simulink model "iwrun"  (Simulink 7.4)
settings: Solver=ode45  StartTime=0  StopTime=5  MaxStep=5e-4  RelTol=1e-3
libraries: mrlib x1

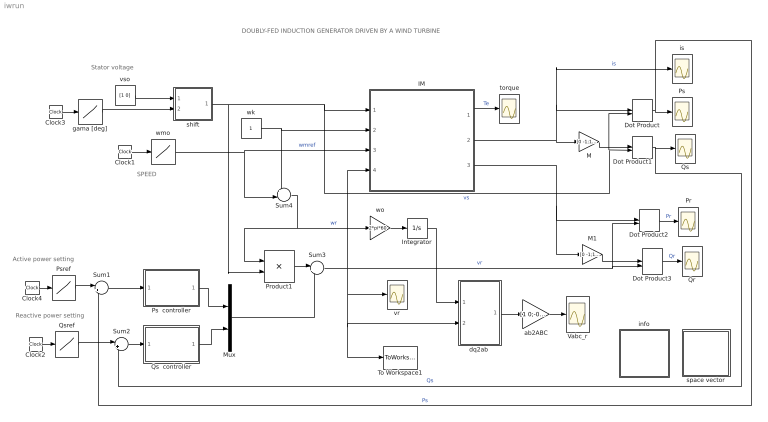
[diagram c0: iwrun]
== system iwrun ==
  note: DOUBLY-FED INDUCTION GENERATOR DRIVEN BY A WIND TURBINE
  note: SPEED
  note: Reactive power setting
  note: Active power setting
  note: Stator voltage
  Clock{1..4} (4 alike) : Clock
  Dot Product{,1..3} (4 alike) : DotProduct  OutDataType=fixdt(1, 16)  OutScaling=2^-10
  IM : Subsystem  mask{Rs=0.01, Lsl=0.1, Rr=0.02, Lm=5, Lrl=0.1, wo=2*pi*60}
      mask prompts: Rs "Stator resistance [pu]"; Lsl "Stator leakage inductance [pu]"; Rr "Rotor resistance [pu]"; Lm "Magnetizing inductance [pu]"; Lrl "Rotor leakage inductance [pu]"; wo "base frequency [rad/s]"
  Integrator : Integrator
  M : Gain  Gain=[0 -1;1 0]  Multiplication=Matrix(K*u)  ParameterDataType=sfix(16)  ParameterScaling=2^0  OutDataType=sfix(16)  OutScaling=2^0
  M1 : Gain  Gain=[0 -1;1 0]  Multiplication=Matrix(K*u)  ParameterDataType=sfix(16)  ParameterScaling=2^0  OutDataType=sfix(16)  OutScaling=2^0
  Mux : Mux  Inputs=2
  Pr : Scope
  Product1 : Product  OutDataType=sfix(16)  OutScaling=2^0
  Ps : Scope
  Ps  controller : Subsystem  mask{Kp=.1, Ki=10, sat=3}
      mask prompts: Kp "Proportional gain (Kp)"; Ki "Integral gain (Ki)"; sat "Saturation limit [pu]"
      mask help: Proportional-Integral Speed Controller
  Psref : Lookup  InputValues=[0 2 2.01 10 ]  Table=[0 0 -1 -1]  OutDataType=sfix(16)  OutScaling=2^0
  Qr : Scope
  Qs : Scope
  Qs  controller : Subsystem  mask{Kp=.1, Ki=10, sat=1000}
      mask prompts: Kp "Proportional gain (Kp)"; Ki "Integral gain (Ki)"; sat "Saturation limit [pu]"
      mask help: Proportional-Integral Speed Controller
  Qsref : Lookup  InputValues=[0 3 3.01 30 ]  Table=[0 0 .5 .5]  OutDataType=sfix(16)  OutScaling=2^0
  Sum1 : Sum  Inputs=|+-  OutDataType=sfix(16)  OutScaling=2^0
  Sum2 : Sum  Inputs=|++  OutDataType=sfix(16)  OutScaling=2^0
  Sum3 : Sum  Inputs=|+-  OutDataType=sfix(16)  OutScaling=2^0
  Sum4 : Sum  Inputs=+-|  OutDataType=sfix(16)  OutScaling=2^0
  To Workspace1 : ToWorkspace  VariableName=vro  SampleTime=-1  SaveFormat=Array
  Vabc_r : Scope
  ab2ABC : Gain  Gain=[1 0;-0.5 sqrt(3)/2;-0.5 -sqrt(3)/2]  Multiplication=Matrix(K*u)  ParameterDataType=sfix(16)  ParameterScaling=2^0  OutDataType=sfix(16)  OutScaling=2^0
  "dq2ab " : Subsystem
  gama [deg] : Lookup  InputValues="[0  1 1.01 5]"  Table=[0 0 10 10]  OutDataType=sfix(16)  OutScaling=2^0
  info : Subsystem
  is : Scope
  shift : Subsystem
  space vector : Subsystem
  torque : Scope
  vr : Scope
  vso : Constant  Value=[1 0]  OutDataType=sfix(16)  OutScaling=2^0
  wk : Constant  OutDataType=sfix(16)  OutScaling=2^0
  wmo : Lookup  InputValues=[0 4 4.01 20 ]  Table=[.7 .7 1.3 1.3]  OutDataType=sfix(16)  OutScaling=2^0
  wo : Gain  Gain=2*pi*60  ParameterDataType=sfix(16)  ParameterScaling=2^0  OutDataType=sfix(16)  OutScaling=2^0
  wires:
  shift/1(vs) -> IM/1(vs), Dot Product/2, Dot Product1/2, Product1/2  "vs"
  wk/1 -> IM/2(wk), Sum4/1
  Dot Product/1 -> Ps/1, Sum1/2  "Ps"
  M/1 -> Dot Product1/1
  Dot Product1/1 -> Qs/1, Sum2/2  "Qs"
  IM/2(is) -> M/1, Dot Product/1, is/1  "is"
  Dot Product2/1 -> Pr/1  "Pr"
  M1/1 -> Dot Product3/1
  Dot Product3/1 -> Qr/1  "Qr"
  IM/3(ir) -> M1/1, Dot Product2/1
  Clock1/1 -> wmo/1
  wmo/1 -> IM/3(wm), Sum4/2  "wmref"
  IM/1(Te) -> torque/1  "Te"
  Qs  controller/1(Vsqer) -> Mux/2
  Sum2/1 -> Qs  controller/1(Qser)
  Sum1/1 -> Ps  controller/1(Pser)
  Ps  controller/1(Vsder) -> Mux/1
  Sum4/1 -> Product1/1, wo/1  "wr"
  Product1/1 -> Sum3/1
  Sum3/1 -> IM/4(vr), Dot Product3/2, Dot Product2/2, vr/1, "dq2ab "/2(dq), To Workspace1/1  "vr"
  Clock4/1 -> Psref/1
  Psref/1 -> Sum1/1
  Clock2/1 -> Qsref/1
  Qsref/1 -> Sum2/1
  Clock3/1 -> gama [deg]/1
  vso/1 -> shift/1(vso)
  gama [deg]/1 -> shift/2(gama)
  "dq2ab "/1(ab) -> ab2ABC/1
  ab2ABC/1 -> Vabc_r/1
  wo/1 -> Integrator/1
  Integrator/1 -> "dq2ab "/1(thetar)
  Mux/1 -> Sum3/2

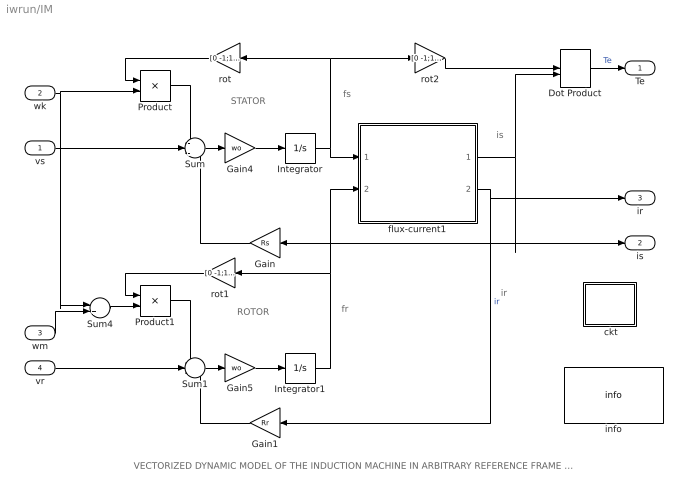
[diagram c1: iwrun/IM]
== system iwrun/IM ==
  note: ROTOR
  note: STATOR
  note: fs
  note: fr
  note: is
  note: VECTORIZED DYNAMIC MODEL OF THE INDUCTION MACHINE IN ARBITRARY REFERENCE FRAME (per unit formulation)
  note: ir
  vs : Inport  OutDataType=sfix(16)  OutScaling=2^0
  wk : Inport  Port=2  OutDataType=sfix(16)  OutScaling=2^0
  wm : Inport  Port=3  OutDataType=sfix(16)  OutScaling=2^0
  vr : Inport  Port=4  OutDataType=sfix(16)  OutScaling=2^0
  " ckt" : Subsystem
  Dot Product : DotProduct  OutDataType=fixdt(1, 16)  OutScaling=2^-10
  Gain : Gain  Gain=Rs  ParameterDataType=sfix(16)  ParameterScaling=2^0  OutDataType=sfix(16)  OutScaling=2^0
  Gain1 : Gain  Gain=Rr  ParameterDataType=sfix(16)  ParameterScaling=2^0  OutDataType=sfix(16)  OutScaling=2^0
  Gain4 : Gain  Gain=wo  ParameterDataType=sfix(16)  ParameterScaling=2^0  OutDataType=sfix(16)  OutScaling=2^0
  Gain5 : Gain  Gain=wo  ParameterDataType=sfix(16)  ParameterScaling=2^0  OutDataType=sfix(16)  OutScaling=2^0
  Integrator : Integrator  InitialCondition=[0 -1]
  Integrator1 : Integrator  InitialCondition=[0 -1]
  Product : Product  OutDataType=sfix(16)  OutScaling=2^0
  Product1 : Product  OutDataType=sfix(16)  OutScaling=2^0
  Sum : Sum  Inputs=-+-  OutDataType=sfix(16)  OutScaling=2^0
  Sum1 : Sum  Inputs=-+-  OutDataType=sfix(16)  OutScaling=2^0
  Sum4 : Sum  Inputs=|+-  OutDataType=sfix(16)  OutScaling=2^0
  flux-current1 : Subsystem
  info : mrlib/IM/info  SystemSampleTime=-1
  rot : Gain  Gain=[0 -1;1 0]  Multiplication=Matrix(K*u)  ParameterDataType=sfix(16)  ParameterScaling=2^0  OutDataType=sfix(16)  OutScaling=2^0
  rot1 : Gain  Gain=[0 -1;1 0]  Multiplication=Matrix(K*u)  ParameterDataType=sfix(16)  ParameterScaling=2^0  OutDataType=sfix(16)  OutScaling=2^0
  rot2 : Gain  Gain=[0 -1;1 0]  Multiplication=Matrix(K*u)  ParameterDataType=sfix(16)  ParameterScaling=2^0  OutDataType=sfix(16)  OutScaling=2^0
  Te : Outport
  is : Outport  Port=2
  ir : Outport  Port=3
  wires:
  Gain/1 -> Sum/3
  Gain1/1 -> Sum1/3
  flux-current1/2(ir) -> Gain1/1, ir/1  "ir"
  Integrator/1 -> flux-current1/1(fs), rot/1, rot2/1
  Integrator1/1 -> flux-current1/2(fr), rot1/1
  Product1/1 -> Sum1/1
  rot1/1 -> Product1/1
  Product/1 -> Sum/1
  rot/1 -> Product/1
  rot2/1 -> Dot Product/1
  Sum4/1 -> Product1/2
  Sum/1 -> Gain4/1
  Gain4/1 -> Integrator/1
  Sum1/1 -> Gain5/1
  Gain5/1 -> Integrator1/1
  flux-current1/1(is) -> Gain/1, is/1, Dot Product/2
  Dot Product/1 -> Te/1  "Te"
  vs/1 -> Sum/2
  wk/1 -> Product/2, Sum4/1
  wm/1 -> Sum4/2
  vr/1 -> Sum1/2

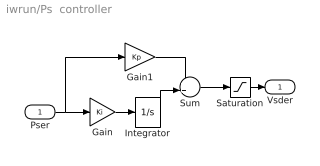
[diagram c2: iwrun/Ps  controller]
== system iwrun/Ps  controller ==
  Pser : Inport  OutDataType=sfix(16)  OutScaling=2^0
  Gain : Gain  Gain=Ki  ParameterDataType=sfix(16)  ParameterScaling=2^0  OutDataType=sfix(16)  OutScaling=2^0
  Gain1 : Gain  Gain=Kp  ParameterDataType=sfix(16)  ParameterScaling=2^0  OutDataType=sfix(16)  OutScaling=2^0
  Integrator : Integrator  LimitOutput=on  UpperSaturationLimit=sat  LowerSaturationLimit=-sat
  Saturation : Saturate  UpperLimit=sat  LowerLimit=-sat
  Sum : Sum  OutDataType=sfix(16)  OutScaling=2^0
  Vsder : Outport  InitialOutput=0
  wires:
  Integrator/1 -> Sum/2
  Gain1/1 -> Sum/1
  Gain/1 -> Integrator/1
  Pser/1 -> Gain/1, Gain1/1
  Sum/1 -> Saturation/1
  Saturation/1 -> Vsder/1

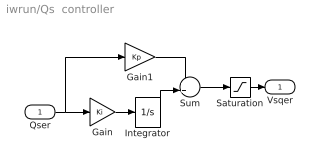
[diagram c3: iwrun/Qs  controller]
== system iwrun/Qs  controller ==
  Qser : Inport  OutDataType=sfix(16)  OutScaling=2^0
  Gain : Gain  Gain=Ki  ParameterDataType=sfix(16)  ParameterScaling=2^0  OutDataType=sfix(16)  OutScaling=2^0
  Gain1 : Gain  Gain=Kp  ParameterDataType=sfix(16)  ParameterScaling=2^0  OutDataType=sfix(16)  OutScaling=2^0
  Integrator : Integrator  LimitOutput=on  UpperSaturationLimit=sat  LowerSaturationLimit=-sat
  Saturation : Saturate  UpperLimit=sat  LowerLimit=-sat
  Sum : Sum  OutDataType=sfix(16)  OutScaling=2^0
  Vsqer : Outport  InitialOutput=0
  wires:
  Saturation/1 -> Vsqer/1
  Sum/1 -> Saturation/1
  Qser/1 -> Gain1/1, Gain/1
  Gain/1 -> Integrator/1
  Gain1/1 -> Sum/1
  Integrator/1 -> Sum/2

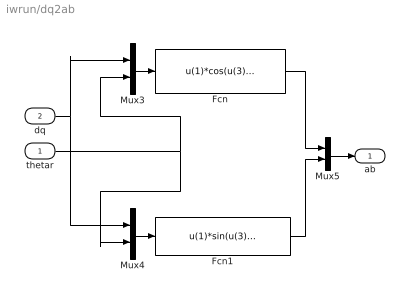
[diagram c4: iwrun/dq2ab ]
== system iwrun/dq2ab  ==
  thetar : Inport  OutDataType=sfix(16)  OutScaling=2^0
  dq : Inport  Port=2  OutDataType=sfix(16)  OutScaling=2^0
  Fcn : Fcn  Expr=u(1)*cos(u(3))-u(2)*sin(u(3))
  Fcn1 : Fcn  Expr=u(1)*sin(u(3))+u(2)*cos(u(3))
  Mux3 : Mux  Inputs=2
  Mux4 : Mux  Inputs=2
  Mux5 : Mux  Inputs=2
  ab : Outport
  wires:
  Mux3/1 -> Fcn/1
  Mux4/1 -> Fcn1/1
  dq/1 -> Mux3/1, Mux4/1
  thetar/1 -> Mux3/2, Mux4/2
  Fcn1/1 -> Mux5/2
  Fcn/1 -> Mux5/1
  Mux5/1 -> ab/1

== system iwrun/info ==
  note: Doubly-Fed Induction Generator driven by a Wind Turbine
  note: The induction machine is modeled in vectorized form in the synchronous frame . The d-axis is aligned with the stator space voltage vector. The injected rotor voltages (at slip frequency) are derived from PI controllers that regulate the active and reactive powers delivered by the generator. The speed is adjusted by the turbine pitch control to maximize the power generated at a given wind speed. The whole system is described by parameters expressed in per unit. The machine representations are based on the motor convention; consequently in the generator mode of operation, such quantities as Ps, Qs, Tw, Te are negative (with wm>0) while Pr is positive for subsynchronous operation and negative for oversynchronous mode.

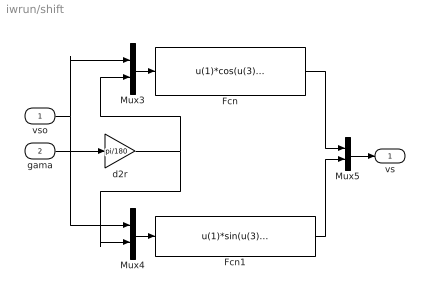
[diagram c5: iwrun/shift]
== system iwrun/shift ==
  vso : Inport  OutDataType=sfix(16)  OutScaling=2^0
  gama : Inport  Port=2  OutDataType=sfix(16)  OutScaling=2^0
  Fcn : Fcn  Expr=u(1)*cos(u(3))-u(2)*sin(u(3))
  Fcn1 : Fcn  Expr=u(1)*sin(u(3))+u(2)*cos(u(3))
  Mux3 : Mux  Inputs=2
  Mux4 : Mux  Inputs=2
  Mux5 : Mux  Inputs=2
  d2r : Gain  Gain=pi/180  Multiplication=Matrix(K*u)  ParameterDataType=sfix(16)  ParameterScaling=2^0  OutDataType=sfix(16)  OutScaling=2^0
  vs : Outport
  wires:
  Mux5/1 -> vs/1
  Fcn/1 -> Mux5/1
  Fcn1/1 -> Mux5/2
  gama/1 -> d2r/1
  vso/1 -> Mux4/1, Mux3/1
  Mux4/1 -> Fcn1/1
  Mux3/1 -> Fcn/1
  d2r/1 -> Mux4/2, Mux3/2

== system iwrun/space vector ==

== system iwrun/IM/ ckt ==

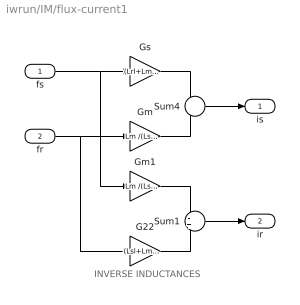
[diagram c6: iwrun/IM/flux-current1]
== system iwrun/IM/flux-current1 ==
  note: INVERSE INDUCTANCES
  fs : Inport  OutDataType=sfix(16)  OutScaling=2^0
  fr : Inport  Port=2  OutDataType=sfix(16)  OutScaling=2^0
  G22 : Gain  Gain=(Lsl+Lm )/(Lsl*Lrl+Lsl*Lm+Lrl*Lm)  ParameterDataType=sfix(16)  ParameterScaling=2^0  OutDataType=sfix(16)  OutScaling=2^0
  Gm : Gain  Gain=Lm /(Lsl*Lrl+Lsl*Lm+Lrl*Lm)  ParameterDataType=sfix(16)  ParameterScaling=2^0  OutDataType=sfix(16)  OutScaling=2^0
  Gm1 : Gain  Gain=Lm /(Lsl*Lrl+Lsl*Lm+Lrl*Lm)  ParameterDataType=sfix(16)  ParameterScaling=2^0  OutDataType=sfix(16)  OutScaling=2^0
  Gs : Gain  Gain=(Lrl+Lm) /(Lsl*Lrl+Lsl*Lm+Lrl*Lm)  ParameterDataType=sfix(16)  ParameterScaling=2^0  OutDataType=sfix(16)  OutScaling=2^0
  Sum1 : Sum  Inputs=-+  OutDataType=sfix(16)  OutScaling=2^0
  Sum4 : Sum  Inputs=+-  OutDataType=sfix(16)  OutScaling=2^0
  is : Outport
  ir : Outport  Port=2
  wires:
  fs/1 -> Gs/1, Gm1/1
  Gs/1 -> Sum4/1
  fr/1 -> Gm/1, G22/1
  Gm/1 -> Sum4/2
  Sum4/1 -> is/1
  Gm1/1 -> Sum1/1
  G22/1 -> Sum1/2
  Sum1/1 -> ir/1
